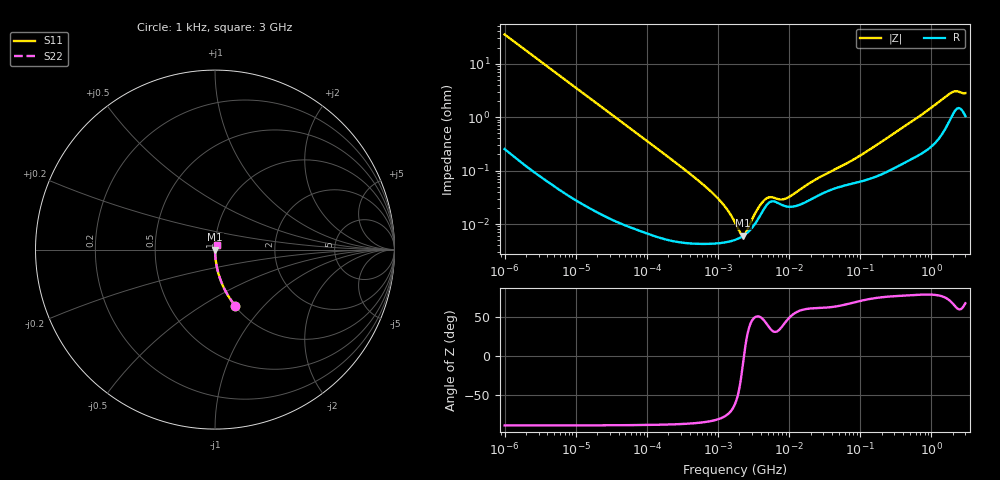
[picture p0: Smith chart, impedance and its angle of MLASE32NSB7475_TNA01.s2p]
! MLASE32NSB7475_TNA01  S-PARAMETER MODEL  ( Standard Model )
! Model Generated by TAIYO YUDEN Corporation (http://www.ty-top.com)
! Version 1.0
! TAIYO YUDEN Control No. 220601
! Copyright(c) 2009 TAIYO YUDEN CO.,LTD. All Rights Reserved.
! Product Description (link to TY-COMPAS)
! https://ds.yuden.co.jp/TYCOMPAS/or/detail?pn=MLASE32NSB7475KTNA01&u=M
! Products Name : Multilayer Ceramic Capacitors
! Characteristics :
!  Capacitance : 4.7 [uF] , Rated Voltage : 16 [V] , TCC : X7R
!  Case Size : 3.2 x 2.5 / 0.126 x 0.098 [mm/inch] , Thickness : 1.9 / 0.075 [mm/inch]
!  (Conditions: Temperature = 25 [degC] , DC Bias Voltage = 0 [V])
! External Node Assignments :
!  1  o---| |---o  2
! GND o---------o GND
! Frequency Range : 1kHz  -  3GHz  [ 401 STEP ]
# MHZ S RI R 50
! Freq[MHz].  S11 Real  S11 Imag  S21 Real  S21 Imag  S12 Real  S12 Imag  S22 Real  S22 Imag
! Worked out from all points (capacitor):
!   401 points, 1 kHz to 3 GHz, reference 50 ohm
!   read as one part in series: C = 4.52 uF near 1.077 kHz
!   lowest |Z| = 6.05 mohm at 2.249 MHz (marker M1)
!   series resonance near 2.317 MHz, so ESL is about 1 nH
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0.001  0.1119 -0.3117  0.8881 0.3117  0.8881 0.3117  0.1119 -0.3117
0.001685  0.0432 -0.1999  0.9568 0.1999  0.9568 0.1999  0.0432 -0.1999
0.00306  0.0139 -0.1138  0.9861 0.1138  0.9861 0.1138  0.0139 -0.1138
0.01216  0.00109 -0.0292  0.9989 0.0292  0.9989 0.0292  0.00109 -0.0292
0.147855  6.17e-05 -0.00243  0.9999 0.00243  0.9999 0.00243  6.17e-05 -0.00243
0.821683  4.29e-05 -0.000387  1 0.000387  1 0.000387  4.29e-05 -0.000387
1.238299  4.52e-05 -0.000212  1 0.000212  1 0.000212  4.52e-05 -0.000212
1.732051  5.04e-05 -9.46e-05  0.9999 9.46e-05  0.9999 9.46e-05  5.04e-05 -9.46e-05
1.866149  5.24e-05 -7.01e-05  0.9999 7.01e-05  0.9999 7.01e-05  5.24e-05 -7.01e-05
2.24859  5.97e-05 -9.68e-06  0.9999 9.68e-06  0.9999 9.68e-06  5.97e-05 -9.68e-06
2.812335  7.67e-05 6.45e-05  0.9999 -6.45e-05  0.9999 -6.45e-05  7.67e-05 6.45e-05
3.789741  0.000134 0.000164  0.9999 -0.000164  0.9999 -0.000164  0.000134 0.000164
4.739869  0.000219 0.000202  0.9998 -0.000202  0.9998 -0.000202  0.000219 0.000202
5.502215  0.000262 0.000181  0.9997 -0.000181  0.9997 -0.000181  0.000262 0.000181
7.414467  0.000237 0.000164  0.9998 -0.000164  0.9998 -0.000164  0.000237 0.000164
8.933959  0.000215 0.000208  0.9998 -0.000208  0.9998 -0.000208  0.000215 0.000208
21.06097  0.000297 0.000548  0.9997 -0.000548  0.9997 -0.000548  0.000297 0.000548
83.67817  0.000587 0.00155  0.9994 -0.00155  0.9994 -0.00155  0.000587 0.00155
256.0921  0.00101 0.00422  0.999 -0.00422  0.999 -0.00422  0.00101 0.00422
1847.629  0.00981 0.0259  0.9902 -0.0259  0.9902 -0.0259  0.00981 0.0259
2226.275  0.0145 0.0264  0.9855 -0.0264  0.9855 -0.0264  0.0145 0.0264
3000  0.0111 0.0256  0.9889 -0.0256  0.9889 -0.0256  0.0111 0.0256
